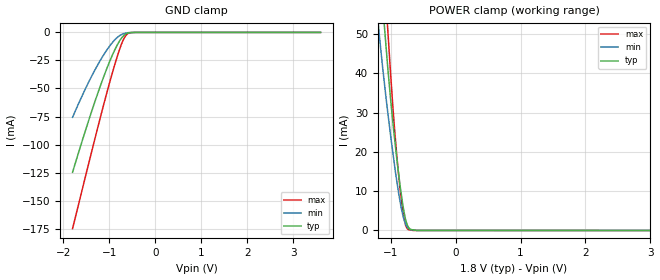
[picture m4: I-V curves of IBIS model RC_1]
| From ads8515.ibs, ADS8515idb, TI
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|   R_C INPUT Model  1.8V
[Model] RC_1
Model_type Input
Vinl = 0.8
Vinh = 1.08
|   typ   min   max
C_comp   7.6429900e-12   6.7918740e-12  8.3793010e-12
[Voltage Range]   1.8   1.65   2
[Temperature Range]   27   85   -40
[Power Clamp Reference]   1.8   1.65   2
[GND Clamp Reference]   0   0   0
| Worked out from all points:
|   GND clamp passes 1 mA (typ) near -0.62 V on its own axis
|   POWER clamp passes 1 mA (typ) near -0.73 V on its own axis
[GND Clamp]
|   Voltage   I  typ   I  min   I  max
-1.8V     -124.7mA   -75.71mA   -174.9mA
-1.614V   -99.82mA   -58.49mA   -144.1mA
-1.376V   -69.35mA   -38.38mA   -105mA
-1.231V   -51.83mA   -27.37mA   -81.45mA
-1.059V   -32.69mA   -16.02mA   -54.6mA
-933.2mV  -20.21mA   -9.063mA   -35.98mA
-789.8mV  -8.518mA   -3.242mA   -16.72mA
-708.6mV  -3.828mA   -1.413mA   -7.743mA
-672.9mV  -2.354mA   -890.4uA   -4.758mA
-610.4mV  -794.8uA   -377.7uA   -1.488mA
-434.6mV  -9.5uA     -9.497uA   -8.839uA
3.595V    0A         0A         0A
[POWER Clamp]
|   Voltage   I  typ   I  min   I  max
-1.8V     224.9mA    179.5mA    278.6mA
-1.183V   71.28mA    51.11mA    90.16mA
-1.092V   51.02mA    36.78mA    64.11mA
-1.044V   41.4mA     30.05mA    51.07mA
-970mV    28.2mA     20.28mA    32.38mA
-937.8mV  23.1mA     16.26mA    25.33mA
-861.7mV  12.28mA    8.001mA    11.54mA
-796.2mV  4.976mA    2.872mA    3.167mA
-764.9mV  2.476mA    1.409mA    1.097mA
-728.4mV  890.3uA    554.4uA    223.6uA
-604.5mV  9.09uA     23.83uA    5.645uA
3.595V    0A         0A         0A
